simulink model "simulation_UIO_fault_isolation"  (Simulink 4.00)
settings: Solver=VariableStepDiscrete  StartTime=0.0  StopTime=ts  RelTol=1e-3
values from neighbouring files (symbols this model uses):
  A = [0.9944 -0.1203 -0.4302    [process_model02.m]
  Auio1 = F1    [UIO_KF_designs.m]
  Auio2 = F2    [UIO_KF_designs.m]
  B = [1 0    [process_model02.m]
  Buio1 = [T1*B K1]    [UIO_KF_designs.m]
  Buio2 = [T2*B K2]    [UIO_KF_designs.m]
  C = [1 0 0    [process_model02.m]
  Cuio1 = eye(3)    [UIO_KF_designs.m]
  Cuio2 = eye(3)    [UIO_KF_designs.m]
  D = zeros(2,2)    [process_model02.m]
  Duio1 = [zeros(3,2) H1]    [UIO_KF_designs.m]
  Duio2 = [zeros(3,2) H2]    [UIO_KF_designs.m]
  x0 = [0.01 0.02 0.03]    [process_model02.m]
undefined symbols (not defined in the file or in its folder): Tc
libraries: simulink3 x2

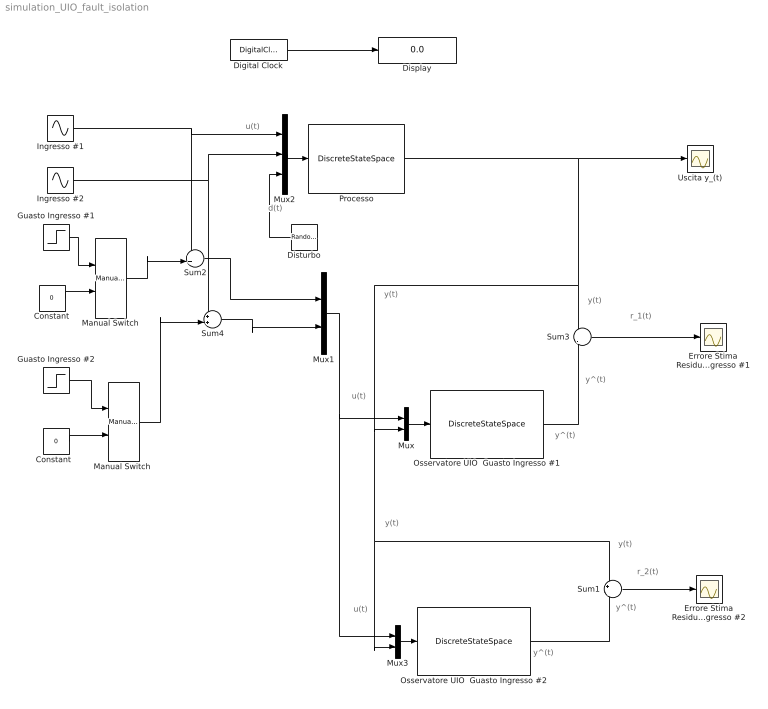
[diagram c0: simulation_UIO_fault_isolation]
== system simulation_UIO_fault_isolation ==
  note: u(t)
  note: y^(t)
  note: y(t)
  note: y^(t)
  note: y^(t)
  note: y^(t)
  note: y(t)
  note: d(t)
  note: u(t)
  note: u(t)
  note: y(t)
  note: y(t)
  note: r_1(t)
  note: r_2(t)
  Constant : Constant  Value=0
  "Constant  " : Constant  Value=0
  Digital Clock : DigitalClock  SampleTime=Tc
  Display : Display
  Disturbo : RandomNumber  Orientation=left  Mean=0  Variance=0.05  Seed=0  SampleTime=Tc
  Errore Stima Residuo Ingresso #1 : Scope
  Errore Stima Residuo Ingresso #2 : Scope
  Guasto Ingresso #1 : Step  Time=25  Before=0  After=1  SampleTime=Tc
  Guasto Ingresso #2 : Step  Time=25  Before=0  After=1  SampleTime=Tc
  Ingresso #1 : Sin  SineType=Time-based  Amplitude=1  Bias=0  Frequency=1  Phase=0  Samples=10  SampleTime=Tc
  Ingresso #2 : Sin  SineType=Time-based  Amplitude=1  Bias=0  Frequency=1  Phase=pi/2  Samples=10  SampleTime=Tc
  Manual Switch : simulink3/Nonlinear/Manual Switch  sw=0  action=0
  "Manual Switch " : simulink3/Nonlinear/Manual Switch  sw=1  action=0
  Mux : Mux  Inputs=2
  Mux1 : Mux  Inputs=2
  Mux2 : Mux  Inputs=3
  Mux3 : Mux  Inputs=2
  Osservatore UIO  Guasto Ingresso #1 : DiscreteStateSpace  A=Auio1  B=Buio1  C=Cuio1  D=Duio1  X0=0  SampleTime=Tc  Realization=auto
  Osservatore UIO  Guasto Ingresso #2 : DiscreteStateSpace  A=Auio2  B=Buio2  C=Cuio2  D=Duio2  X0=0  SampleTime=Tc  Realization=auto
  Processo : DiscreteStateSpace  A=A  B=[B E]  C=C  D=D  X0=x0  SampleTime=Tc  Realization=auto
  Sum1 : Sum  Inputs=+|-  SaturateOnIntegerOverflow=on
  Sum2 : Sum  Inputs=++|  SaturateOnIntegerOverflow=on
  Sum3 : Sum  Inputs=+|-  SaturateOnIntegerOverflow=on
  Sum4 : Sum  Inputs=++|  SaturateOnIntegerOverflow=on
  Uscita y_(t) : Scope
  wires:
  Digital Clock/1 -> Display/1
  Mux2/1 -> Processo/1
  Ingresso #1/1 -> Mux2/1, Sum2/1
  Processo/1 -> Sum3/1, Mux/2, Mux3/2, Sum1/1, Uscita y_(t)/1
  Mux/1 -> Osservatore UIO  Guasto Ingresso #1/1
  Osservatore UIO  Guasto Ingresso #1/1 -> Sum3/2
  Sum3/1 -> Errore Stima Residuo Ingresso #1/1
  Mux3/1 -> Osservatore UIO  Guasto Ingresso #2/1
  Osservatore UIO  Guasto Ingresso #2/1 -> Sum1/2
  Sum1/1 -> Errore Stima Residuo Ingresso #2/1
  Disturbo/1 -> Mux2/3
  Ingresso #2/1 -> Mux2/2, Sum4/1
  Mux1/1 -> Mux/1, Mux3/1
  Sum4/1 -> Mux1/2
  Sum2/1 -> Mux1/1
  Constant/1 -> Manual Switch/2
  Guasto Ingresso #1/1 -> Manual Switch/1
  Manual Switch/1 -> Sum2/2
  "Constant  "/1 -> "Manual Switch "/2
  Guasto Ingresso #2/1 -> "Manual Switch "/1
  "Manual Switch "/1 -> Sum4/2
